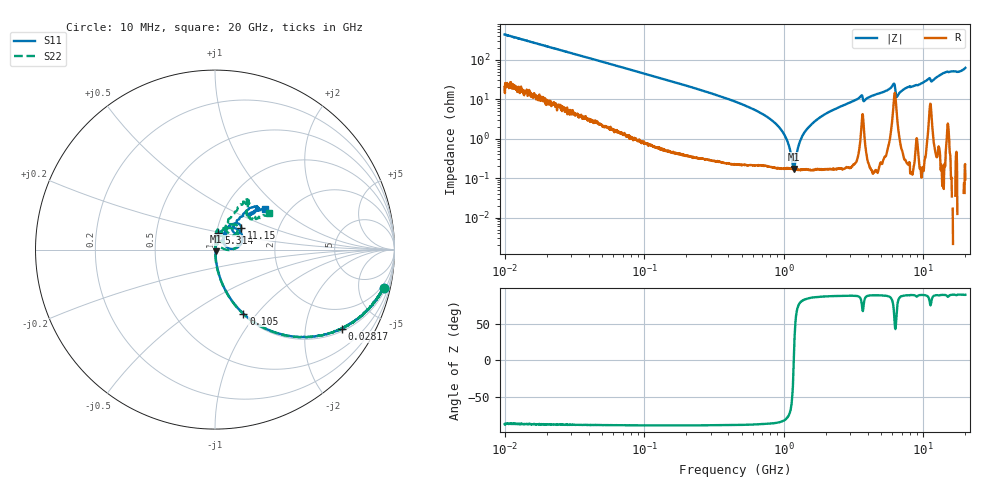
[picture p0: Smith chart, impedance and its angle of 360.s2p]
!Keysight Technologies,P5008B,MY61100088,A.16.20.02
!Date: Friday, August 30, 2024 14:04:29
!Correction: S11(C  2-Port  )
!S21(C  2-Port  )
!S12(C  2-Port  )
!S22(C  2-Port  )
!S2P File: Measurements: S11, S21, S12, S22:Log Frequency Sweep
# Hz S  MA  R 50
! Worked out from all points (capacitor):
!   1601 points, 10 MHz to 20 GHz, reference 50 ohm
!   read as one part in series: C = 36.4 pF near 10.39 MHz
!   lowest |Z| = 170 mohm at 1.179 GHz (marker M1)
!   series resonance near 1.18 GHz, so ESL is about 500 pH
!   S11 on the Smith chart (normalised r, x): 10 MHz: 1.39, -8.74; 28.17 MHz: 1.08, -3.15; 105 MHz: 1.01, -0.85; 5.314 GHz: 1.02, +0.19; 11.15 GHz: 1.30, +0.33; 20 GHz: 1.52, +0.80
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1e7  0.9655 -12.7  0.2206 74.6  0.2205 74.6  0.965 -12.7
2.81686e7  0.8343 -32.0  0.5295 56.5  0.5293 56.5  0.8341 -32.0
3.555162e7  0.7697 -38.0  0.6159 50.2  0.6156 50.3  0.7696 -38.1
1.050162e8  0.3904 -66.0  0.9138 22.8  0.9133 22.8  0.3906 -66.2
1.263918e8  0.3334 -69.7  0.9377 19.3  0.9372 19.3  0.3335 -69.9
4.472136e8  0.09134 -83.2  0.9938 4.8  0.9932 4.7  0.09129 -84.5
8.655496e8  0.03318 -83.5  0.9978 1.0  0.9973 1.0  0.03278 -88.6
1.178681e9  0.01115 -67.7  0.9985 -0.6  0.998 -0.6  0.01045 -96.1
1.359223e9  0.002265 4.6  0.9986 -1.3  0.9981 -1.3  0.0009826 11.4
1.589917e9  0.009832 71.5  0.9986 -2.2  0.9981 -2.2  0.009107 85.3
2.025791e9  0.02567 80.6  0.9985 -3.6  0.998 -3.6  0.02512 83.8
3.53169e9  0.0785 77.4  0.9892 -8.7  0.989 -8.8  0.07785 71.6
3.846973e9  0.05713 83.3  0.993 -7.9  0.9927 -8.0  0.05779 67.6
5.313894e9  0.09542 78.2  0.9933 -12.8  0.9929 -12.9  0.09745 70.8
5.652411e9  0.1063 73.0  0.989 -14.2  0.9886 -14.3  0.1085 69.6
6.098795e9  0.1612 48.6  0.9311 -17.2  0.9306 -17.3  0.1516 49.7
6.611766e9  0.05951 37.7  0.9847 -12.3  0.9842 -12.4  0.04404 77.4
7.697294e9  0.1062 59.5  0.9958 -17.1  0.9953 -17.3  0.1033 80.9
9.30816e9  0.1047 56.7  0.9963 -21.4  0.9957 -21.6  0.1029 74.6
1.11497e10  0.1914 39.9  0.9257 -27.2  0.9251 -27.5  0.1666 40.8
1.413906e10  0.3173 48.1  0.9601 -35.3  0.9598 -35.5  0.3135 58.0
2e10  0.3611 39.2  0.9364 -53.2  0.9365 -53.6  0.3641 33.8
